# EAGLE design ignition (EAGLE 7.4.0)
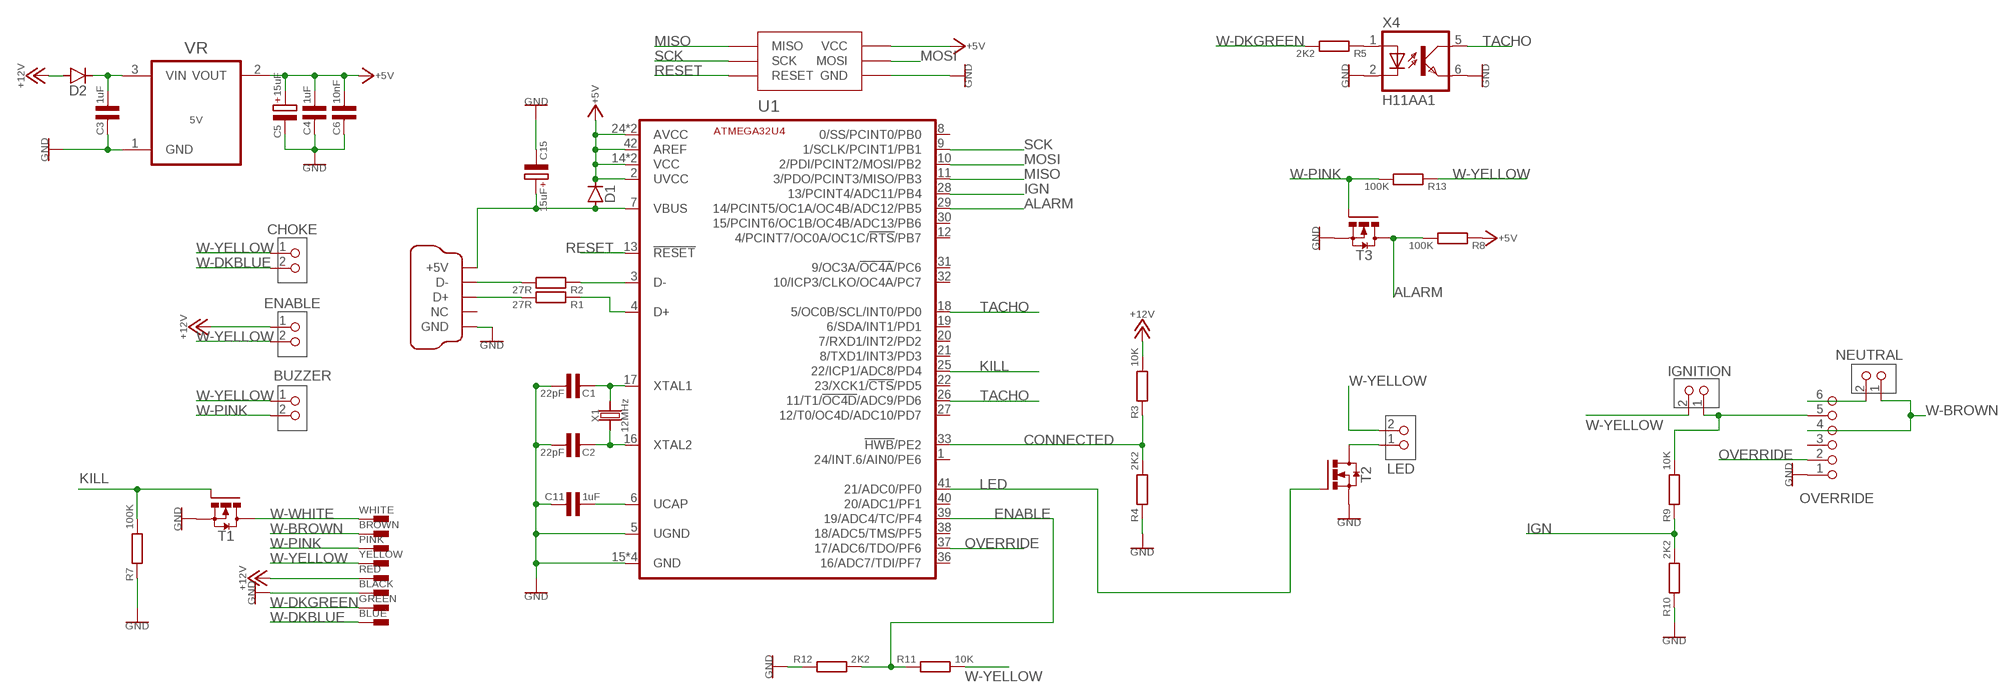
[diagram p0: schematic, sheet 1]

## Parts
BLACK  FASTONF061.100  [FASTON-6.3MM]
BLUE  FASTONF061.100  [FASTON-6.3MM]
BROWN  FASTONF061.100  [FASTON-6.3MM]
BUZZER  PINHD-1X2MOLEXKK  [1X02/MOLEXKK]
C1  22pF  C-EU0603  [0603]
C2  22pF  C-EU0603  [0603]
C3  1uF  C-EU0603  [0603]
C4  1uF  C-EU0603  [0603]
C5  15uF  CAPACITOR-POLARISEDEIA3216  [EIA3216]
C6  10nF  C-EU0603  [0603]
C11  1uF  C-EU0603  [0603]
C15  15uF  CAPACITOR-POLARISEDEIA3216  [EIA3216]
CHOKE  PINHD-1X2MOLEXKK  [1X02/MOLEXKK]
D1  DIODE0603  [0603-DIODE]
D2  DIODE0603  [0603-DIODE]
ENABLE  PINHD-1X2MOLEXKK  [1X02/MOLEXKK]
GREEN  FASTONF061.100  [FASTON-6.3MM]
IGNITION  PINHD-1X2MOLEXKK  [1X02/MOLEXKK]
LED  PINHD-1X2MOLEXKK  [1X02/MOLEXKK]
NEUTRAL  PINHD-1X2MOLEXKK  [1X02/MOLEXKK]
OVERRIDE  PINHD-1X6MOLEX-KK  [1X06/MOLEXKK]
PINK  FASTONF061.100  [FASTON-6.3MM]
R1  27R  R-EU0603  [0603]
R2  27R  R-EU0603  [0603]
R3  10K  R-EU0603  [0603]
R4  2K2  R-EU0603  [0603]
R5  2K2  R-EU0603  [0603]
R7  100K  R-EU0603  [0603]
R8  100K  R-EU0603  [0603]
R9  10K  R-EU0603  [0603]
R10  2K2  R-EU0603  [0603]
R11  10K  R-EU0603  [0603]
R12  2K2  R-EU0603  [0603]
R13  100K  R-EU0603  [0603]
RED  FASTONF061.100  [FASTON-6.3MM]
T1  BSS138  MOSFET-NCHSOT-23  [SOT23]
T2  BSS138  MOSFET-NCHSOT-23  [SOT23]
T3  BSS138  MOSFET-NCHSOT-23  [SOT23]
U1  ATMEGA32U4  [QFN44]
U$1  AVRISPTAG-CONNECT  [TAG-CONNECT-2030NL]
VR  5V  MCP1703SOT23  [SOT23]
WHITE  FASTONF061.100  [FASTON-6.3MM]
X1  12MHz  CRYSTAL3.2X2.5MM  [CRYSTAL-3.2X2.5MM]
X2  MINI-USB  [MINI-USB]
X4  H11AA1  OPTOCOUPLERDIP6  [DIP6-SM]
YELLOW  FASTONF061.100  [FASTON-6.3MM]

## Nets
+5V: C4.1 C5.+ C6.1 D1.1(K) R8.1 U1.2(UVCC) U1.14(VCC) U1.24(AVCC) U1.34(VCC) U1.42(AREF) U1.44(AVCC) U$1.2(VCC) VR.2(VOUT)
+12V: D2.2(A) ENABLE.1 R3.2 RED.A1 RED.A2
ALARM: R8.2 T3.3(D) U1.29(14/PCINT5/OC1A/OC4B/ADC12/PB5)
CONNECTED: R3.1 R4.2 U1.33(!HWB!/PE2)
ENABLE: R11.1 R12.2 U1.39(19/ADC4/TC/PF4)
GND: BLACK.A1 BLACK.A2 C1.1 C2.1 C3.2 C4.2 C5.- C6.2 C11.2 C15.- OVERRIDE.1 R4.1 R7.1 R10.1 R12.1 T1.2(S) T2.2(S) T3.2(S) U1.5(UGND) U1.15(GND) U1.23(GND) U1.35(GND) U1.43(GND) U$1.6(GND) VR.1(GND) X2.5(GND) X4.2(C) X4.6(EMIT)
IGN: R9.1 R10.2 U1.28(13/PCINT4/ADC11/PB4)
KILL: R7.2 T1.1(G) U1.25(22/ICP1/ADC8/PD4)
LED: T2.1(G) U1.41(21/ADC0/PF0)
MISO: U1.11(3/PDO/PCINT3/MISO/PB3) U$1.1(MISO)
MOSI: U1.10(2/PDI/PCINT2/MOSI/PB2) U$1.4(MOSI)
N$1: C2.2 U1.16(XTAL2) X1.1
N$2: C1.2 U1.17(XTAL1) X1.3
N$3: R5.1 X4.1(A)
N$4: R2.2 X2.2(D-)
N$6: R2.1 U1.3(D-)
N$7: R1.1 U1.4(D+)
N$8: R1.2 X2.3(D+)
N$9: C11.1 U1.6(UCAP)
N$10: IGNITION.1 OVERRIDE.5 R9.2
N$11: LED.1 T2.3(D)
N$14: C3.1 D2.1(K) VR.3(VIN)
N$15: NEUTRAL.2 OVERRIDE.6
OVERRIDE: OVERRIDE.2 U1.37(17/ADC6/TDO/PF6)
RESET: U1.13(!RESET!) U$1.5(RESET)
SCK: U1.9(1/SCLK/PCINT1/PB1) U$1.3(SCK)
TACHO: U1.18(5/OC0B/SCL/INT0/PD0) U1.26(11/T1/!OC4D!/ADC9/PD6) X4.5(COL)
VBUS: C15.+ D1.2(A) U1.7(VBUS) X2.1(+5V)
W-BROWN: BROWN.A1 BROWN.A2 NEUTRAL.1 OVERRIDE.4
W-DKBLUE: BLUE.A1 BLUE.A2 CHOKE.2
W-DKGREEN: GREEN.A1 GREEN.A2 R5.2
W-PINK: BUZZER.2 PINK.A1 PINK.A2 R13.2 T3.1(G)
W-WHITE: T1.3(D) WHITE.A1 WHITE.A2
W-YELLOW: BUZZER.1 CHOKE.1 ENABLE.2 IGNITION.2 LED.2 R11.2 R13.1 YELLOW.A1 YELLOW.A2
Unconnected: OVERRIDE.3 U1.1(24/INT.6/AIN0/PE6) U1.8(0/SS/PCINT0/PB0) U1.12(4/PCINT7/OC0A/OC1C/!RTS!/PB7) U1.19(6/SDA/INT1/PD1) U1.20(7/RXD1/INT2/PD2) U1.21(8/TXD1/INT3/PD3) U1.22(23/XCK1/!CTS!/PD5) U1.27(12/T0/OC4D/ADC10/PD7) U1.30(15/PCINT6/OC1B/OC4B/ADC13/PB6) U1.31(9/OC3A/!OC4A!/PC6) U1.32(10/ICP3/CLKO/OC4A/PC7) U1.36(16/ADC7/TDI/PF7) U1.38(18/ADC5/TMS/PF5) U1.40(20/ADC1/PF1) X2.4(NC)

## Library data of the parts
BLACK BLUE BROWN GREEN PINK RED WHITE YELLOW = MikesParts:FASTON: Faston tab; OC_FARNELL: unknown; OC_NEWARK: unknown
BUZZER CHOKE ENABLE IGNITION LED NEUTRAL = MikesParts:PINHD-1X2: PIN HEADER
C1-C4 C6 C11 = MikesParts:C-EU
C5 C15 = MikesParts:CAPACITOR-POLARISED: Polarised Capacitor
D1 D2 = MikesParts:DIODE
OVERRIDE = MikesParts:PINHD-1X6: PIN HEADER
R1-R5 R7-R13 = MikesParts:R-EU: resistor
T1-T3 = MikesParts:MOSFET-NCH: MOSFET N-Channel, eg BSS138, BUK7Y13, FDN335N
U1 = MikesParts:ATMEGA32U4
U$1 = MikesParts:AVRISP
VR = MikesParts:MCP1703: IC REG LDO 250MA: 2V5, 3V3, 5V0
X1 = MikesParts:CRYSTAL
X2 = MikesParts:MINI-USB: MINI USB-B Conector Source: www.cypressindustries.com
X4 = MikesParts:OPTOCOUPLER: Opto isolator, eg PC354N, H11AA1 or SFH628 (latter two have bidirectional LEDs)

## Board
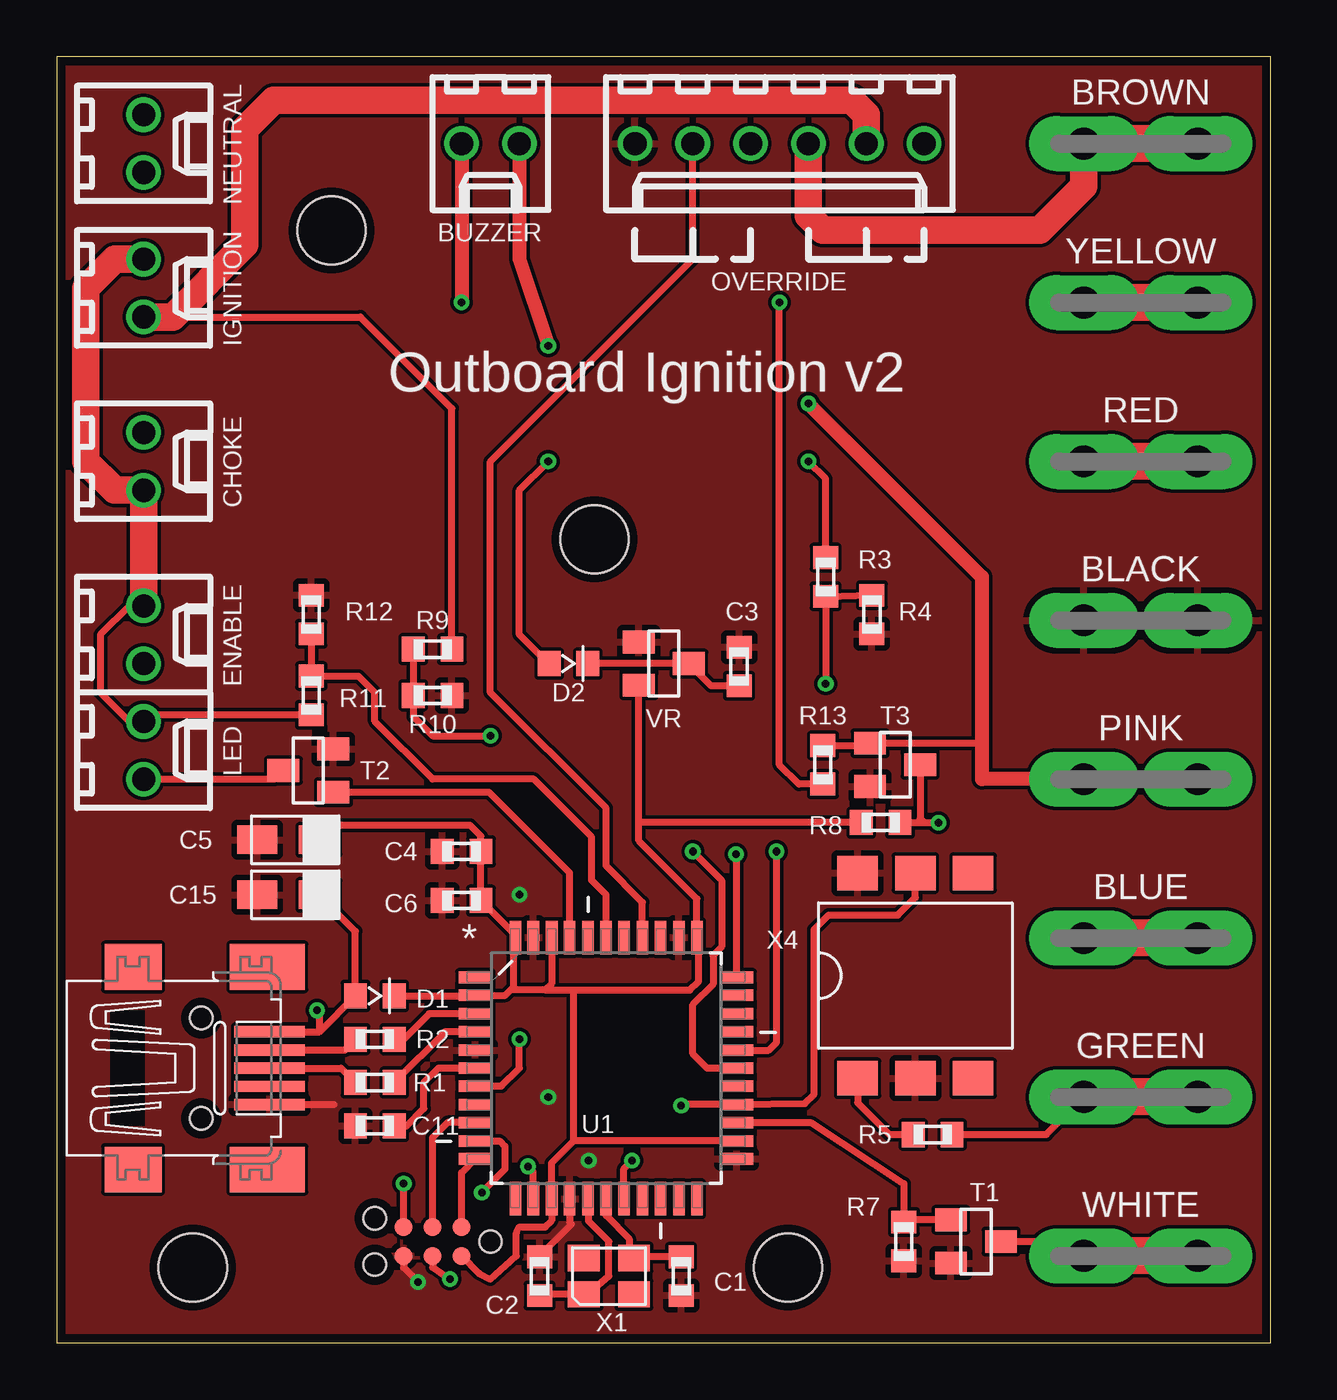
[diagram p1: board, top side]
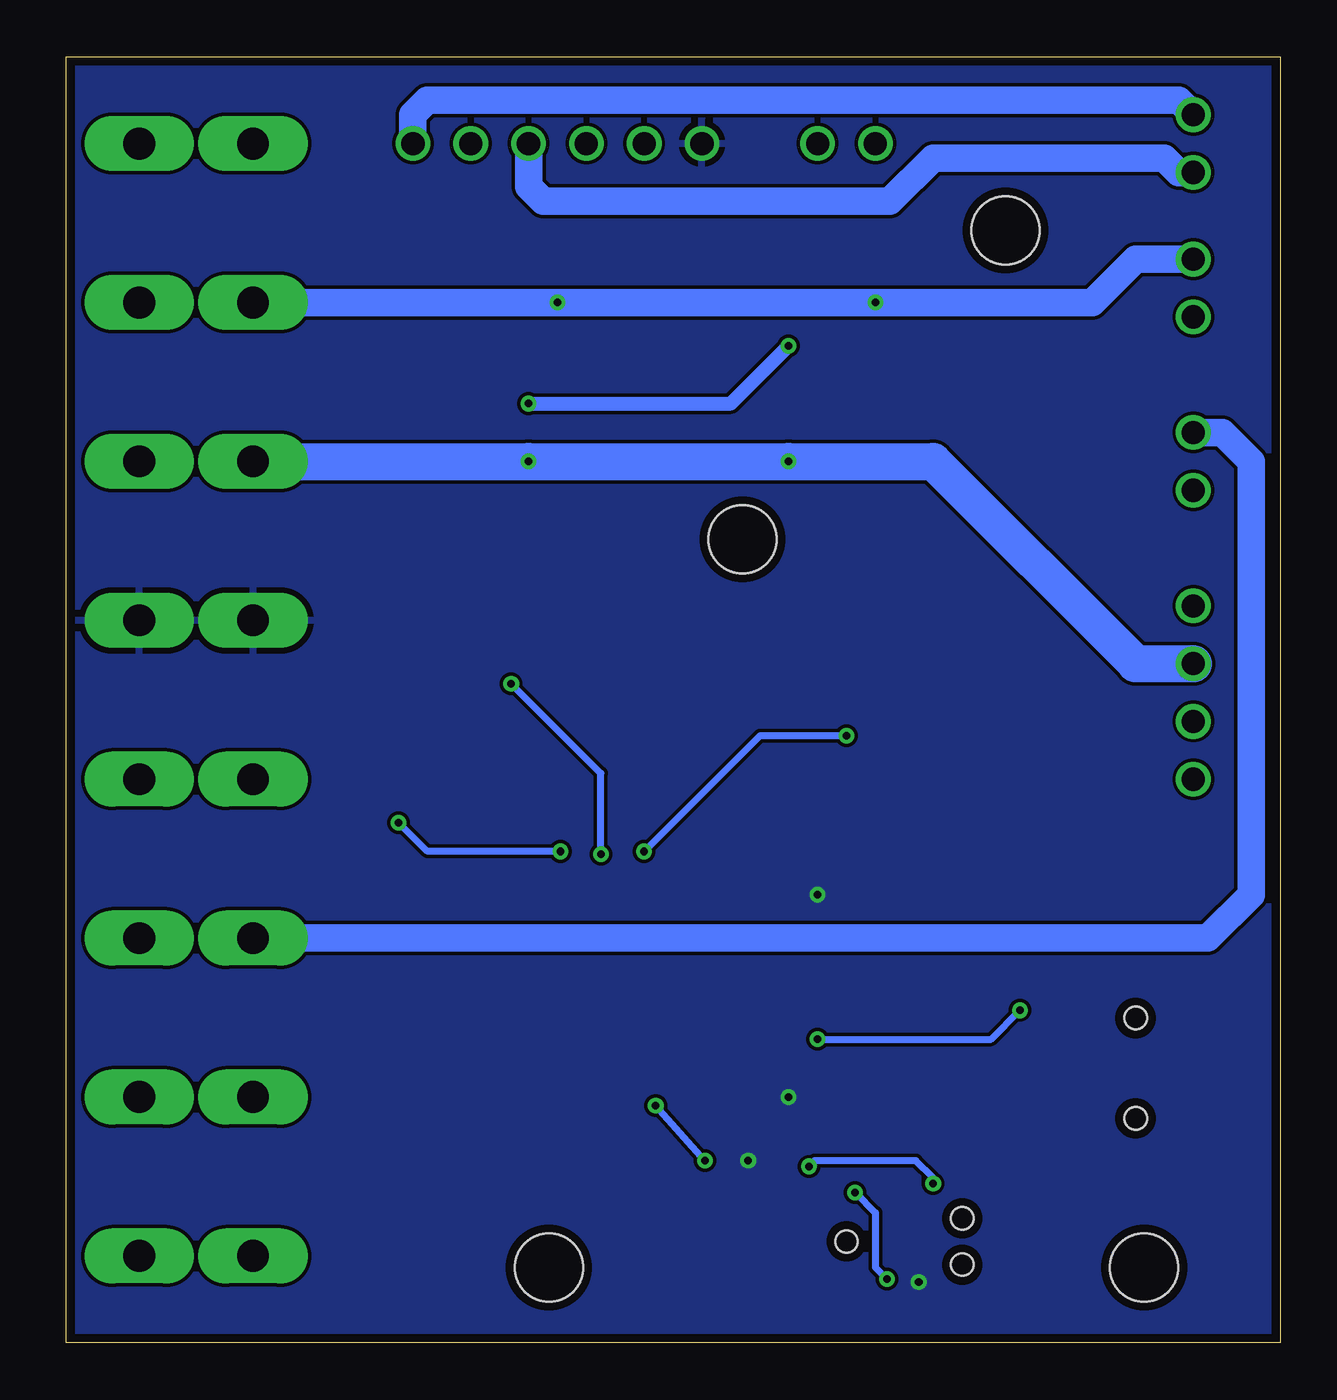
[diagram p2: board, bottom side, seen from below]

Size 53.34 x 56.52 mm. Coordinates in mm from the lower left corner, seen from the top.
Outline: 0,0 53.34,0 53.34,56.52 0,56.52 0,0
Copper layers (1*16): Top 0.0356mm / dielectric 1.5011mm / Bottom 0.0356mm
Design rules "LaenPCBOrder-maskvia": minimum track width 6mil, minimum drill 13mil, track to track 6mil, track to pad 6mil, pad to pad 6mil, via to via 6mil, smd to smd 6mil, copper to edge 15mil, drill to drill 6mil, minimum pad ring 7mil, minimum via ring 7mil, stop-mask expansion 4mil, vias tented up to drill 13mil, thermal gap 10mil
Holes 3 mm at 12.06,48.9 5.97,3.3 32.13,3.3 23.62,35.31

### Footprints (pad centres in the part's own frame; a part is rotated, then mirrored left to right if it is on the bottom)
FASTON-6.3MM = drill 1.4 pad 2.413 long: A1 -2.5,0; A2 2.5,0
1X02/MOLEXKK = drill 1.016: 1 -1.27,0; 2 1.27,0
0603 = smd 1 x 1.1: 1 -0.85,0; 2 0.85,0
EIA3216 = smd 1.75 x 1.25: + -1.35,0; - 1.35,0
0603-DIODE = smd 1 x 1.1: 1 -0.85,0; 2 0.85,0
1X06/MOLEXKK = drill 1.016: 1 -6.35,0; 2 -3.81,0; 3 -1.27,0; 4 1.27,0; 5 3.81,0; 6 6.35,0
SOT23 = smd 1.4 x 1: 1 -1.1,0.95; 2 -1.1,-0.95; 3 1.1,0
QFN44 = smd 1.473 x 0.508: 1 -5.74,3.988; 2 -5.74,3.2; 3 -5.74,2.388; 4 -5.74,1.6; 5 -5.74,0.787; 6 -5.74,0; 7 -5.74,-0.787; 8 -5.74,-1.6; 9 -5.74,-2.388; 10 -5.74,-3.2; 11 -5.74,-3.988; 23 5.74,-3.988; 24 5.74,-3.2; 25 5.74,-2.388; 26 5.74,-1.6; 27 5.74,-0.787; 28 5.74,0; 29 5.74,0.787; 30 5.74,1.6; 31 5.74,2.388; 32 5.74,3.2; 33 5.74,3.988 | smd 0.508 x 1.473: 12 -3.988,-5.74; 13 -3.2,-5.74; 14 -2.388,-5.74; 15 -1.6,-5.74; 16 -0.787,-5.74; 17 0,-5.74; 18 0.787,-5.74; 19 1.6,-5.74; 20 2.388,-5.74; 21 3.2,-5.74; 22 3.988,-5.74; 34 3.988,5.74; 35 3.2,5.74; 36 2.388,5.74; 37 1.6,5.74; 38 0.787,5.74; 39 0,5.74; 40 -0.787,5.74; 41 -1.6,5.74; 42 -2.388,5.74; 43 -3.2,5.74; 44 -3.988,5.74
TAG-CONNECT-2030NL = smd 0.787 x 0.787: 1 -1.27,-0.635; 2 -1.27,0.635; 3 0,-0.635; 4 0,0.635; 5 1.27,-0.635; 6 1.27,0.635 | hole 0.991: -2.54,0; 2.54,1.016; 2.54,-1.016
CRYSTAL-3.2X2.5MM = smd 1.15 x 1.4: 1 -0.8,1.1; 2 -0.8,-1.1; 3 0.8,-1.1; 4 0.8,1.1
MINI-USB = smd 3.1 x 0.5: 1 3,1.6; 2 3,0.8; 3 3,0; 4 3,-0.8; 5 3,-1.6 | smd 2.5 x 2: M1 -3,-4.45; M2 -3,4.45 | smd 3.3 x 2: M3 2.9,4.45; M4 2.9,-4.45 | hole 1: 0,2.2; 0,-2.2
DIP6-SM = smd 1.52 x 1.78: 1 -4.51,2.54; 2 -4.51,0; 3 -4.51,-2.54; 4 4.51,-2.54; 5 4.51,0; 6 4.51,2.54

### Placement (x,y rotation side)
BLACK  47.62,31.75 0 top
BLUE  47.62,17.78 0 top
BROWN  47.62,52.7 0 top
BUZZER  19.05,52.7 0 top
C1  27.43,2.92 90 top
C2  21.21,2.92 270 top
C3  29.97,29.72 90 top
C4  17.78,21.59 180 top
C5  10.16,22.1 180 top
C6  17.78,19.43 180 top
C11  13.97,9.53 180 top
C15  10.16,19.68 180 top
CHOKE  3.81,38.73 90 top
D1  13.97,15.24 180 top
D2  22.48,29.84 180 top
ENABLE  3.81,31.11 90 top
GREEN  47.62,10.79 0 top
IGNITION  3.81,46.35 90 top
LED  3.81,26.04 90 top
NEUTRAL  3.81,52.7 90 top
OVERRIDE  31.75,52.7 0 top
PINK  47.62,24.77 0 top
R1  13.97,11.43 180 top
R2  13.97,13.34 180 top
R3  33.78,33.66 90 top
R4  35.81,32 90 top
R5  38.48,9.14 0 top
R7  37.21,4.45 90 top
R8  36.2,22.86 0 top
R9  16.51,30.48 0 top
R10  16.51,28.45 180 top
R11  11.18,28.45 270 top
R12  11.18,32 270 top
R13  33.66,25.4 90 top
RED  47.62,38.73 0 top
T1  40.39,4.45 0 top
T2  11.05,25.15 180 top
T3  36.83,25.4 0 top
U1  24.13,12.06 0 top
U$1  16.51,4.45 180 top
VR  26.67,29.84 0 top
WHITE  47.62,3.81 0 top
X1  24.26,2.92 90 top
X2  6.35,12.06 0 top
X4  37.72,16.13 90 top
YELLOW  47.62,45.72 0 top

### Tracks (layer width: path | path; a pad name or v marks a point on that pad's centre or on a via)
+5V
  Top 0.305: D1.1 18.36,15.24 U1.2 19.71,15.27 19.94,15.49 | U$1.2 18.54,3.05 19.05,2.79 20.19,3.81 20.19,4.83 20.32,5.08 21.46,5.08 21.74,5.36 U1.14 21.74,7.9 22.71,8.87 | U1.24 22.71,8.87 | 19.94,15.49 20.07,15.62 20.07,17.73 U1.44 20.14,17.92 C6.1 C4.1 18.63,22.26 18.16,22.73 12.14,22.73 C5.+ | U1.42 21.74,15.77 21.46,15.49 | 21.46,15.49 19.94,15.49 | 21.46,15.49 22.73,15.49 | 22.73,15.49 27.81,15.49 28.19,15.88 28.19,17.73 U1.34 28.12,19.51 25.57,22.05 25.57,22.86 | 25.57,22.86 VR.2 | 22.71,8.87 22.71,15.47 22.73,15.49 | R8.1 25.57,22.86
+12V  (via drill 0.33)
  Top 0.305: D2.2 21.59,29.84 20.32,31.11 20.32,37.47 v21.59,38.73 | R3.2 33.78,37.97 v33.02,38.73
  Top 1.626: RED.A2 RED.A1
  Bottom 1.626: RED.A1 v33.02,38.73 v21.59,38.73 15.24,38.73 6.35,29.84 ENABLE.1
ALARM  (via drill 0.33)
  Top 0.305: U1.29 31.27,12.85 31.62,13.21 v31.62,21.59 | R8.2 38.1,22.86 | 38.1,22.86 v38.73,22.86 | T3.3 37.93,23.03 38.1,22.86
  Bottom 0.305: v31.62,21.59 37.47,21.59 v38.73,22.86
CONNECTED  (via drill 0.33)
  Top 0.305: U1.33 29.87,21.44 v29.84,21.46 | v33.78,28.96 R3.1 R4.2
  Bottom 0.305: v29.84,21.46 29.84,25.02 v33.78,28.96
ENABLE
  Top 0.305: R12.2 R11.1 13.25,29.3 13.97,28.57 13.97,27.3 16.51,24.77 20.95,24.77 23.5,22.23 23.5,20.32 24.13,19.68 U1.39
GND  (via drill 0.33)
  Top 0.305: X2.5 12.18,10.46 | C2.1 21.17,3.77 22.61,5.21 22.53,5.28 U1.15 | U$1.6 15.24,3.3 v15.88,2.67
  other vias: 21.59,10.79 20.32,19.68 23.37,8
  pour Top: 0,0 53.34,0 53.34,56.52 0,56.52
  pour Bottom: 0,0 53.34,0 53.34,56.39 0,56.39
IGN  (via drill 0.33)
  Top 0.305: R9.1 R10.2 15.66,27.52 16.51,26.67 v19.05,26.67 | v27.94,21.59 29.21,20.32 29.21,17.4 28.83,17.02 28.83,15.75 27.94,14.86 27.94,12.7 28.57,12.06 U1.28
  Bottom 0.305: v19.05,26.67 22.86,26.67 v27.94,21.59
KILL
  Top 0.305: T1.1 37.49,5.39 R7.2 37.21,6.99 33.12,9.68 U1.25
LED
  Top 0.305: T2.1 18.98,24.2 22.53,20.65 U1.41
MISO
  Top 0.305: U$1.1 17.78,7.47 U1.11
MOSI  (via drill 0.33)
  Top 0.305: U$1.4 16.51,3.3 v17.27,2.79 | U1.10 19.46,8.87 19.68,8.64 19.68,7.62 v18.67,6.6
  Bottom 0.305: v18.67,6.6 17.78,5.71 17.78,3.3 v17.27,2.79
N$1
  Top 0.305: U1.16 23.37,6.3 23.37,5.33 24.26,4.45 24.26,2.92 23.33,2.12 X1.1 21.13,2.12 C2.2
N$2
  Top 0.305: U1.17 24.13,5.59 25.15,4.57 25.15,4.06 X1.3 25.28,3.77 C1.2
N$3
  Top 0.305: X4.1 35.18,10.54 36.58,9.14 R5.1
N$4
  Top 0.305: X2.2 12.65,12.87 R2.2
N$6
  Top 0.305: U1.3 16.36,14.45 15.24,13.34 R2.1
N$7
  Top 0.305: U1.4 17.05,13.66 R1.1
N$8
  Top 0.305: X2.3 12.48,12.06 R1.2
N$9
  Top 0.305: C11.1 15.37,9.53 16.13,10.29 16.13,11.43 16.76,12.06 U1.6
N$10
  Top 0.305: 5.08,45.09 13.34,45.09 17.36,41.06 R9.2
  Top 1.219: OVERRIDE.5 35.56,53.98 34.92,54.61 9.53,54.61 8.26,53.34 8.26,48.26 5.08,45.09 IGNITION.1
N$11
  Top 0.305: LED.1 9.57,24.77 T2.3
N$14
  Top 0.305: C3.1 28.75,28.87 VR.3 D2.1
N$15
  Bottom 1.219: NEUTRAL.2 4.45,54.61 37.47,54.61 38.1,53.98 OVERRIDE.6
OVERRIDE
  Top 0.305: U1.37 25.73,19.36 24.13,20.95 24.13,23.5 19.05,28.57 19.05,38.73 27.94,47.62 OVERRIDE.2
RESET  (via drill 0.33)
  Top 0.305: U$1.5 v15.24,6.99 | U1.13 20.93,7.52 v20.7,7.75
  Bottom 0.305: v15.24,6.99 15.24,7.24 16,8 20.45,8 v20.7,7.75
SCK
  Top 0.305: U1.9 17.17,9.68 16.51,9.02 U$1.3
TACHO  (via drill 0.33)
  Top 0.305: X4.5 37.72,19.56 36.96,18.8 33.91,18.8 33.27,18.16 33.27,10.92 32.87,10.52 U1.26 27.48,10.46 v27.43,10.41 | U1.18 24.92,7.64 v25.27,8
  Bottom 0.305: v25.27,8 v27.43,10.41
VBUS  (via drill 0.33)
  Top 0.305: X2.1 11.54,13.66 | 11.54,13.66 D1.2 13.12,18.07 C15.+ | U1.7 19.53,11.28 20.32,12.06 v20.32,13.34 | 11.54,13.66 11.54,14.49 v11.43,14.61
  Bottom 0.305: v20.32,13.34 12.7,13.34 v11.43,14.61
W-BROWN
  Top 1.219: BROWN.A1 45.12,50.84 43.18,48.9 33.66,48.9 33.02,49.53 OVERRIDE.4
  Top 1.626: BROWN.A2 BROWN.A1
  Bottom 1.219: NEUTRAL.1 4.45,51.44 5.08,52.07 15.24,52.07 17.14,50.16 32.38,50.16 33.02,50.8 OVERRIDE.4
W-DKBLUE
  Top 1.626: BLUE.A2 BLUE.A1
  Bottom 1.219: BLUE.A1 3.17,17.78 1.27,19.68 1.27,38.73 2.54,40.01 CHOKE.2
W-DKGREEN
  Top 0.305: R5.2 43.47,9.14 GREEN.A1
  Top 1.626: GREEN.A2 GREEN.A1 44.45,10.79
W-PINK  (via drill 0.33)
  Top 0.305: R13.2 35.63,26.25 T3.1 40.57,26.35 40.64,26.42
  Top 0.61: v33.02,41.27 40.64,33.66 40.64,26.42 40.64,24.77 PINK.A1 PINK.A2 | BUZZER.2 20.32,47.62 v21.59,43.81
  Bottom 0.61: v33.02,41.27 24.13,41.27 v21.59,43.81
W-WHITE
  Top 0.305: T1.3 44.62,4.45 WHITE.A1
  Top 1.626: WHITE.A2 WHITE.A1
W-YELLOW  (via drill 0.33)
  Top 0.305: R11.2 4.1,27.6 LED.2 3.17,27.3 1.91,28.57 1.91,31.11 3.17,32.38 ENABLE.2 | R13.1 32.6,24.55 31.75,25.4 v31.75,45.72
  Top 0.61: BUZZER.1 v17.78,45.72
  Top 1.219: ENABLE.2 CHOKE.1 2.54,37.47 1.27,38.73 1.27,46.35 2.54,47.62 IGNITION.2
  Top 1.626: YELLOW.A2 YELLOW.A1
  Bottom 1.219: YELLOW.A1 v31.75,45.72 v17.78,45.72 8.26,45.72 6.35,47.62 IGNITION.2

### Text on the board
tPlace: Outboard Ignition v2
